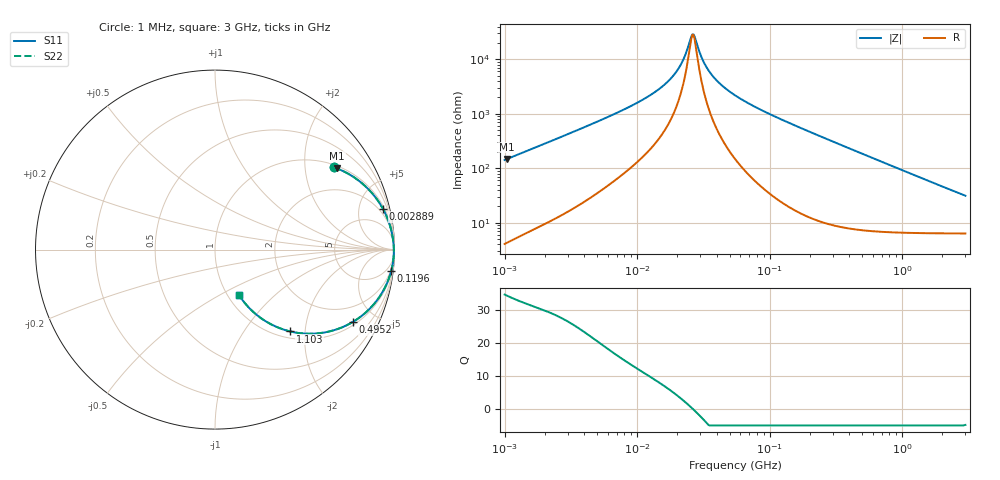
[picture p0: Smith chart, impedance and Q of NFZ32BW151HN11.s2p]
! NFZ32BW151HN11
# Hz S RI R 50
!Freq.(Hz) S11(Real) S11(Imag) S21(Real) S21(Imag) S12(Real) S12(Imag) S22(Real) S22(Imag)
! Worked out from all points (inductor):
!   401 points, 1 MHz to 3 GHz, reference 50 ohm
!   read as one part in series: L = 22.4 uH near 1.041 MHz
!   highest Q = 34.4 at 1.041 MHz (marker M1), where L = 22.5 uH
!   self-resonance near 26.12 MHz
!   S11 on the Smith chart (normalised r, x): 1 MHz: 1.08, +2.83; 2.889 MHz: 1.30, +8.14; 119.6 MHz: 1, -16; 495.2 MHz: 1.15, -3.73; 1.103 GHz: 1.13, -1.67; 3 GHz: 1.13, -0.61
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1000000  0.6634 0.4584  0.3366 -0.4584  0.3366 -0.4584  0.6634 0.4584
1040844  0.6802 0.4521  0.3198 -0.4521  0.3198 -0.4521  0.6802 0.4521
1682724  0.8412 0.3498  0.1588 -0.3498  0.1588 -0.3498  0.8412 0.3498
2888807  0.9356 0.2276  0.0644 -0.2276  0.0644 -0.2276  0.9356 0.2276
3823119  0.9602 0.1757  0.0398 -0.1757  0.0398 -0.1757  0.9602 0.1757
8861669  0.9894 0.0719  0.0106 -0.0719  0.0106 -0.0719  0.9894 0.0719
1.461624e7  0.9945 0.0346  0.00553 -0.0346  0.00553 -0.0346  0.9945 0.0346
2.013356e7  0.996 0.0153  0.00402 -0.0153  0.00402 -0.0153  0.996 0.0153
2.270269e7  0.9963 0.00841  0.00369 -0.00841  0.00369 -0.00841  0.9963 0.00841
2.559965e7  0.9965 0.00163  0.00347 -0.00163  0.00347 -0.00163  0.9965 0.00163
2.664524e7  0.9966 -0.000623  0.00343 0.000623  0.00343 0.000623  0.9966 -0.000623
3.127247e7  0.9966 -0.00972  0.00338 0.00972  0.00338 0.00972  0.9966 -0.00972
3.526298e7  0.9965 -0.0167  0.00348 0.0167  0.00348 0.0167  0.9965 -0.0167
4.22235e7  0.9961 -0.0277  0.00389 0.0277  0.00389 0.0277  0.9961 -0.0277
5.477226e7  0.9948 -0.0453  0.00515 0.0453  0.00515 0.0453  0.9948 -0.0453
1.195584e8  0.9814 -0.1208  0.0186 0.1208  0.0186 0.1208  0.9814 -0.1208
2.094008e8  0.9472 -0.2108  0.0528 0.2108  0.0528 0.2108  0.9472 -0.2108
4.951867e8  0.7678 -0.4031  0.2322 0.4031  0.2322 0.4031  0.7678 -0.4031
8.005644e8  0.5665 -0.4673  0.4335 0.4673  0.4335 0.4673  0.5665 -0.4673
1.10276e9  0.4183 -0.4558  0.5817 0.4558  0.5817 0.4558  0.4183 -0.4558
1.818868e9  0.2334 -0.3645  0.7666 0.3645  0.7666 0.3645  0.2334 -0.3645
3e9  0.1318 -0.2503  0.8682 0.2503  0.8682 0.2503  0.1318 -0.2503
